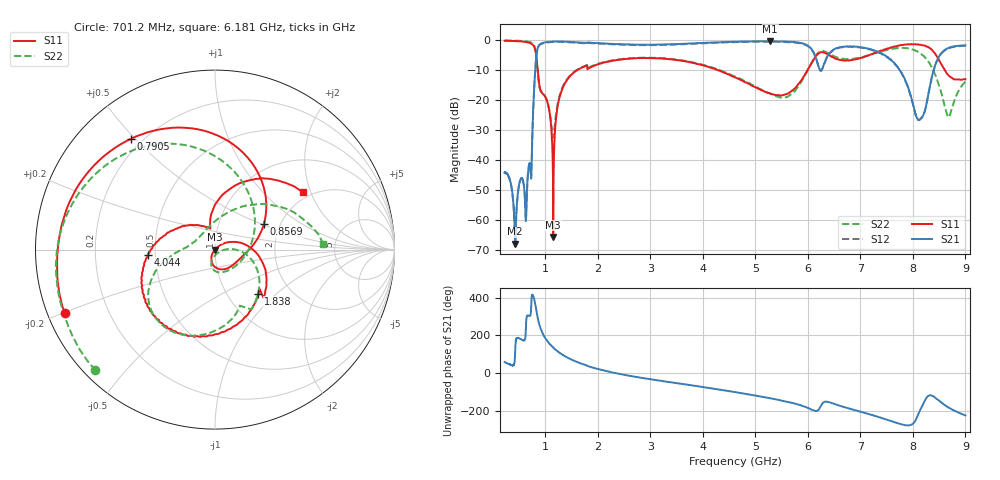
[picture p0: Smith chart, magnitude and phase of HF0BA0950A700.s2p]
!Agilent Technologies,E8358A,US41080443,A.07.50.56
!Agilent E8358A: A.07.50.56
!Date: Wednesday, May 04, 2016 15:26:24
!Correction: S11(Full 2 Port(1,2))
!S21(Full 2 Port(1,2))
!S12(Full 2 Port(1,2))
!S22(Full 2 Port(1,2))
!S2P File: Measurements: S11, S21, S12, S22:Log Frequency Sweep
# Hz S  dB  R 50
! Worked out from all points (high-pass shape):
!   1601 points, 225 MHz to 9 GHz, reference 50 ohm
!   highest |S21| = -0.28 dB at 5.284 GHz (marker M1); lowest = -67.9 dB at 427.1 MHz (marker M2)
!   |S21| within 3 dB of the highest: 846 MHz to 6.084 GHz (5.238 GHz wide, 151 % of centre); 6.473 GHz to 7.261 GHz (788.1 MHz wide, 11.5 % of centre)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
!   lowest |S11| = -65.7 dB at 1.151 GHz (marker M3), VSWR 1.00, Z = 50 - j0.0356 ohm
!   |S11| at or under -10 dB: 855.4 MHz to 1.601 GHz (745.8 MHz wide, 60.7 % of centre); 4.303 GHz to 5.992 GHz (1.688 GHz wide, 32.8 % of centre); 8.612 GHz to end of sweep
!   |S22| runs from -32.4 to 0.0 dB; largest |S21 - S12| = 0.019
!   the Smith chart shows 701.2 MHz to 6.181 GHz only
!   S11 on the Smith chart (normalised r, x): 701.2 MHz: 0.05, -0.20; 790.5 MHz: 0.16, +0.49; 856.9 MHz: 1.65, +0.51; 1.838 GHz: 1.39, -0.78; 4.044 GHz: 0.45, -0.03; 6.181 GHz: 1.80, +1.76
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2.25e8  -0.12 -34.0  -44.13 57.9  -44.23 58.1  -0.01 -29.3
4.271107e8  -0.23 -69.9  -67.87 117.8  -67.65 119.6  -0.09 -60.0
4.996064e8  -0.28 -85.7  -48.21 -175.3  -48.42 -175.4  -0.13 -73.7
6.306059e8  -0.52 -124.5  -60.16 -120.9  -60.57 -119.7  -0.28 -106.8
7.011602e8  -0.82 -157.0  -40.95 -57.3  -41.09 -57.1  -0.47 -134.7
7.904678e8  -2.21 127.2  -15.13 30.4  -15.26 30.5  -1.79 155.3
8.568983e8  -10.28 27.4  -2.50 -68.6  -2.65 -68.4  -10.73 40.7
9.705073e8  -18.15 -59.4  -0.76 -160.8  -0.91 -160.7  -17.96 -82.9
1.15105e9  -65.65 -136.9  -0.36 134.5  -0.51 134.7  -32.39 -44.6
1.279833e9  -18.47 21.1  -0.34 105.5  -0.50 105.7  -17.95 -1.5
1.687749e9  -9.16 -34.6  -0.74 49.6  -0.88 49.7  -9.01 -48.8
1.838042e9  -9.23 -45.6  -0.71 34.0  -0.86 34.2  -8.95 -68.3
3.152512e9  -5.99 -131.4  -1.38 -40.1  -1.54 -40.0  -5.88 -128.5
4.043857e9  -8.51 -175.4  -0.79 -76.8  -0.94 -76.8  -8.36 -156.2
4.622431e9  -12.39 150.2  -0.42 -102.4  -0.57 -102.3  -12.10 -171.7
5.283785e9  -17.75 108.5  -0.28 -134.6  -0.44 -134.7  -17.82 162.5
6.081681e9  -7.25 63.1  -3.22 163.7  -3.37 163.8  -7.20 32.9
6.180629e9  -4.67 33.4  -7.31 158.9  -7.49 158.8  -4.39 3.2
6.562452e9  -6.26 -67.9  -2.49 -170.7  -2.66 -170.9  -5.68 -80.7
7.553438e9  -2.59 -167.9  -6.08 107.1  -6.22 107.0  -3.02 -174.5
8.131784e9  -1.49 138.4  -26.41 159.0  -26.51 159.1  -4.19 66.4
9e9  -12.95 121.8  -1.64 133.9  -1.81 133.9  -13.78 -46.7
